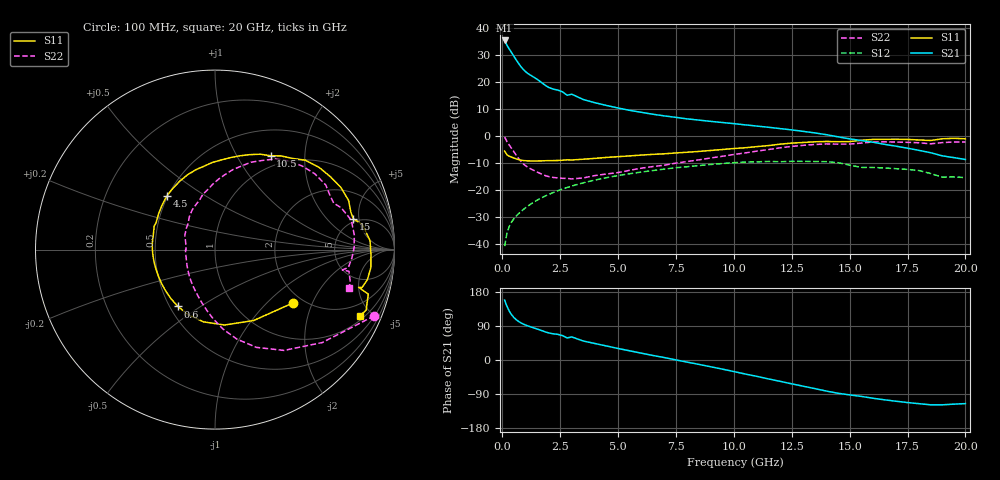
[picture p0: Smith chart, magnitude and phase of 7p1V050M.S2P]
! Infineon Technologies  Discrete & RF Semiconductors
! bfp620
! VCE =  1.0 V,  IC =  50 mA
! Common Emitter S-Parameters:  Sep 2002
# GHz  S  MA  R  50
!  f  S11  S21  S12  S22
! GHz  MAG  ANG  MAG  ANG  MAG  ANG  MAG  ANG
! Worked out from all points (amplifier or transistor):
!   59 points, 100 MHz to 20 GHz, reference 50 ohm
!   highest |S21| = 35.3 dB at 100 MHz (marker M1)
!   |S21| within 3 dB of that: start of sweep to 288.6 MHz
!   unconditionally stable (mu >= 1): 2.667 GHz to 2.926 GHz; 3.177 GHz to 10 GHz; 17.12 GHz to end of sweep
!   at 1 GHz: K = 0.86, MSG = 25.2 dB, |S12| = -26.6 dB
!   at 5.5 GHz: K = 1.04, MAG = 10.5 dB, |S12| = -13.9 dB
!   at 20 GHz: K = 1.39, MAG = -0.4 dB, |S12| = -15.4 dB
!   S11 on the Smith chart (normalised r, x): 100 MHz: 1.77, -1.46; 600 MHz: 0.55, -0.41; 4.5 GHz: 0.49, +0.35; 10.5 GHz: 0.84, +1.39; 15 GHz: 4.61, +4.18; 20 GHz: 1.23, -4.27
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0.1  0.5269 -34.3  58.47 158.0  0.0092 79.8  0.9608 -22.6
0.2  0.45 -61.4  47.81 141.9  0.0159 68.9  0.7908 -40.9
0.3  0.4235 -82.8  40.63 129.2  0.0212 64.9  0.6808 -55.6
0.4  0.4076 -99.0  34.88 119.5  0.0257 62.7  0.5919 -67.0
0.5  0.3925 -112.1  29.9 112.2  0.0295 61.5  0.5132 -76.3
0.6  0.3784 -123.1  25.62 106.5  0.0331 60.8  0.4443 -84.3
0.7  0.3669 -132.4  22.07 101.9  0.0366 60.5  0.3871 -91.3
0.8  0.3585 -140.2  19.27 98.1  0.04 60.3  0.342 -97.6
1  0.3496 -151.9  15.56 92.4  0.047 60.0  0.2831 -108.3
1.3  0.3462 -163.6  12.69 86.0  0.0578 59.3  0.2384 -120.6
1.8  0.3488 -179.7  9.025 75.4  0.0758 56.7  0.1894 -142.9
2  0.3507 174.9  7.94 71.5  0.083 55.3  0.1779 -151.5
2.8  0.3637 158.6  5.677 58.2  0.112 48.7  0.1647 -178.9
3  0.3605 155.9  5.933 60.8  0.1191 46.9  0.1611 -179.3
3.5  0.373 147.1  4.731 50.1  0.1367 42.1  0.1679 166.6
4.5  0.4024 131.7  3.674 37.0  0.1699 32.2  0.1988 143.5
7  0.4696 97.1  2.355 6.4  0.2447 6.6  0.2892 107.3
10.5  0.6078 59.4  1.607 -37.1  0.3297 -33.6  0.4877 72.5
13.5  0.7823 26.3  1.141 -75.5  0.3379 -69.7  0.6979 37.3
15  0.7896 12.5  0.887 -92.1  0.2902 -90.9  0.7104 21.4
17  0.874 -6.6  0.65 -108.8  0.2493 -101.0  0.7754 0.9
20  0.8879 -24.5  0.368 -115.1  0.1703 -111.4  0.776 -16.2
